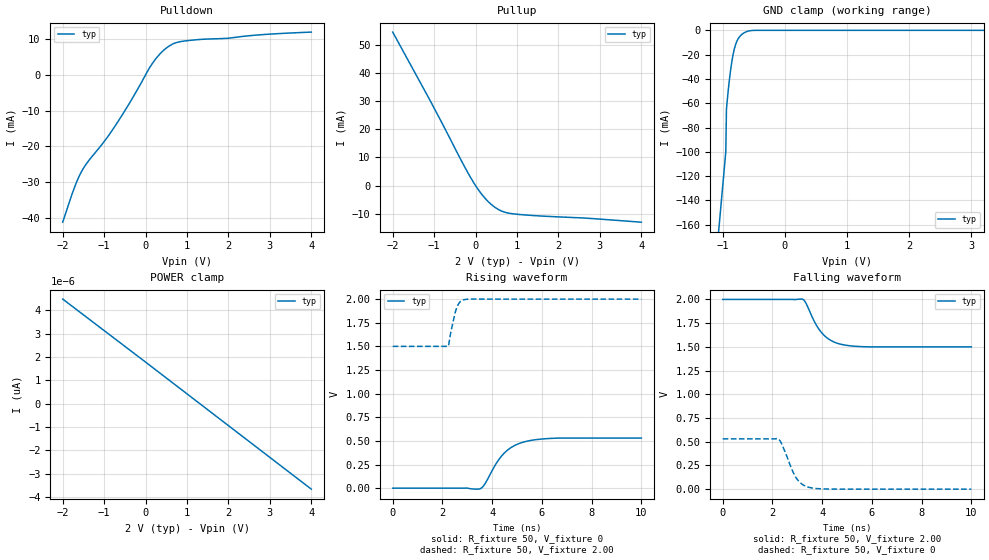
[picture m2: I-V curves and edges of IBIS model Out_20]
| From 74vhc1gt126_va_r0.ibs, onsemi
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|//////////////////////////////////////////////////////////////////////////////
|//////////////////////////////////////////////////////////////////////////////
[Model] Out_20
Model_type 3-state
Polarity Non-Inverting
Enable Active-High
Vmeas = 1.00
Vref = 2.0
Rref = 1k
Cref = 15pF
|  variable   typ   min   max
C_comp   3.8pF   3.8pF   3.8pF
|//////////////////////////////////////////////////////////////////////////////
[Temperature Range]   25   125   -55
|//////////////////////////////////////////////////////////////////////////////
[Voltage Range]   2.00V   NA   NA
|//////////////////////////////////////////////////////////////////////////////
[Pulldown Reference]   0V   NA   NA
|//////////////////////////////////////////////////////////////////////////////
[Pullup Reference]   2.00V   NA   NA
|//////////////////////////////////////////////////////////////////////////////
[GND Clamp Reference]   0V   NA   NA
|//////////////////////////////////////////////////////////////////////////////
[POWER Clamp Reference] 2.00V   NA   NA
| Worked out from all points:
|   slope of the pulldown table from 0 to 0.3 V, typ, clamps not added: 57.5 ohm
|   slope of the pullup table from 0 to 0.3 V, typ, clamps not added: 53.6 ohm
|   GND clamp passes 1 mA (typ) near -0.61 V on its own axis
|   falling waveform, R_fixture 50, V_fixture 2.00: 20-80 % time 714ps typ, NA min, NA max; typ from 2 V to 1.5 V
|   falling waveform, R_fixture 50, V_fixture 0: 20-80 % time 532ps typ, NA min, NA max; typ from 0.53 V to 0 V
|   rising waveform, R_fixture 50, V_fixture 0: 20-80 % time 888ps typ, NA min, NA max; typ from 0 V to 0.53 V
|   rising waveform, R_fixture 50, V_fixture 2.00: 20-80 % time 260ps typ, NA min, NA max; typ from 1.5 V to 2 V
|//////////////////////////////////////////////////////////////////////////////
[Pulldown]
|   Voltage   I(typ)   I(min)   I(max)
-2V       -41.15mA   NA         NA
-1.68V    -30.36mA   NA         NA
-1.52V    -26.46mA   NA         NA
-960mV    -18.03mA   NA         NA
-720mV    -14.02mA   NA         NA
-310mV    -6.395mA   NA         NA
160mV     3.095mA    NA         NA
340mV     5.735mA    NA         NA
520mV     7.628mA    NA         NA
730mV     8.937mA    NA         NA
1.03V     9.556mA    NA         NA
4V        11.92mA    NA         NA
|//////////////////////////////////////////////////////////////////////////////
[Pullup]
|   Voltage   I(typ)   I(min)   I(max)
-2V       54.4mA     NA         NA
-1.11V    30.5mA     NA         NA
-320mV    8.205mA    NA         NA
-120mV    2.884mA    NA         NA
20mV      -448.2uA   NA         NA
160mV     -3.283mA   NA         NA
300mV     -5.595mA   NA         NA
440mV     -7.389mA   NA         NA
680mV     -9.297mA   NA         NA
960mV     -10.08mA   NA         NA
4V        -12.96mA   NA         NA
|//////////////////////////////////////////////////////////////////////////////
[GND Clamp]
|   Voltage   I(typ)   I(min)   I(max)
-2V       -695.6mA   NA         NA
-1.09V    -179.3mA   NA         NA
-1.05V    -156.6mA   NA         NA
-950mV    -99.85mA   NA         NA
-940mV    -65.07mA   NA         NA
-900mV    -44.12mA   NA         NA
-870mV    -31.64mA   NA         NA
-830mV    -19.22mA   NA         NA
-780mV    -9.983mA   NA         NA
-720mV    -4.765mA   NA         NA
-640mV    -1.629mA   NA         NA
4V        4.479pA    NA         NA
|//////////////////////////////////////////////////////////////////////////////
[POWER Clamp]
|   Voltage   I(typ)   I(min)   I(max)
-2V       4.479pA    NA         NA
0V        1.777pA    NA         NA
2V        -945.6fA   NA         NA
4V        -3.668pA   NA         NA
|//////////////////////////////////////////////////////////////////////////////
|//////////////////////////////////////////////////////////////////////////////
[Ramp]
|  variable   typ   min   max
dV/dt_r   3.180E-01/9.000E-10  NA   NA
dV/dt_f   3.000E-01/7.000E-10  NA   NA
R_load = 50
|//////////////////////////////////////////////////////////////////////////////
[Falling Waveform]
R_fixture = 50
V_fixture = 2.00
C_fixture = 0p
|   time   V(typ)   V(min)   V(max)
0s        2V         NA         NA
3.2ns     2.003V     NA         NA
3.35ns    1.96V      NA         NA
3.7ns     1.761V     NA         NA
4ns       1.643V     NA         NA
4.2ns     1.594V     NA         NA
4.4ns     1.561V     NA         NA
4.9ns     1.519V     NA         NA
5.9ns     1.5V       NA         NA
10ns      1.5V       NA         NA
|//////////////////////////////////////////////////////////////////////////////
[Falling Waveform]
R_fixture = 50
V_fixture = 0
C_fixture = 0p
|   time   V(typ)   V(min)   V(max)
0s        530mV      NA         NA
2.225ns   530.3mV    NA         NA
2.3ns     511.4mV    NA         NA
2.375ns   475.4mV    NA         NA
2.775ns   212.4mV    NA         NA
2.95ns    121.9mV    NA         NA
3.2ns     50.94mV    NA         NA
3.525ns   15.92mV    NA         NA
4.5ns     678.4uV    NA         NA
10ns      0V         NA         NA
|//////////////////////////////////////////////////////////////////////////////
[Rising Waveform]
R_fixture = 50
V_fixture = 0
C_fixture = 0p
|   time   V(typ)   V(min)   V(max)
0s        0V         NA         NA
3.5ns     -7.809mV   NA         NA
3.6ns     8.2mV      NA         NA
3.7ns     41.49mV    NA         NA
4.15ns    255.4mV    NA         NA
4.5ns     374.6mV    NA         NA
4.9ns     450.9mV    NA         NA
5.45ns    499.7mV    NA         NA
6.65ns    529.7mV    NA         NA
10ns      530mV      NA         NA
|//////////////////////////////////////////////////////////////////////////////
[Rising Waveform]
R_fixture = 50
V_fixture = 2.00
C_fixture = 0p
|   time   V(typ)   V(min)   V(max)
0s        1.5V       NA         NA
2.225ns   1.499V     NA         NA
2.25ns    1.513V     NA         NA
2.325ns   1.632V     NA         NA
2.475ns   1.815V     NA         NA
2.575ns   1.908V     NA         NA
2.625ns   1.939V     NA         NA
2.7ns     1.968V     NA         NA
2.9ns     1.996V     NA         NA
10ns      2V         NA         NA
